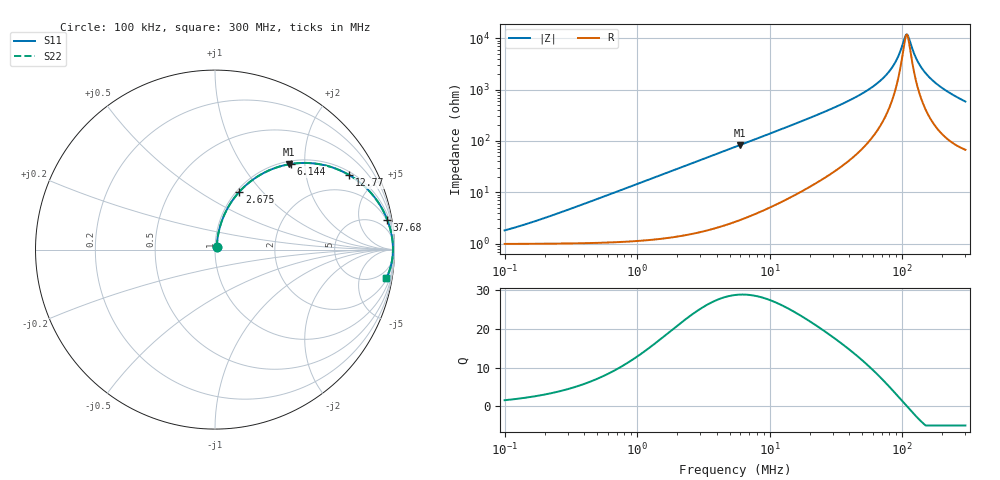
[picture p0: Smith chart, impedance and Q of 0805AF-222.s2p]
# MHz  S  MA  R  50
!Freq  MagS11  AngS11  MagS21  AngS21  MagS12  AngS12  MagS22  AngS22
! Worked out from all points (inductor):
!   801 points, 100 kHz to 300 MHz, reference 50 ohm
!   read as one part in series: L = 2.37 uH near 201.7 kHz
!   highest Q = 28.9 at 5.962 MHz (marker M1), where L = 2.21 uH
!   self-resonance near 107.9 MHz
!   S11 on the Smith chart (normalised r, x): 100 kHz: 1.02, +0.03; 2.675 MHz: 1.03, +0.76; 6.144 MHz: 1.06, +1.71; 12.77 MHz: 1.14, +3.52; 37.68 MHz: 2, +11; 300 MHz: 2, -12
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0.1  0.01791 56.1  0.9901 -0.9  0.9901 -0.9  0.01791 56.1
0.3829105  0.05666 76.6  0.9884 -3.2  0.9884 -3.2  0.05666 76.6
1.451587  0.2013 75.0  0.9677 -11.6  0.9677 -11.6  0.2013 75.0
2.674748  0.3487 67.2  0.9228 -20.4  0.9228 -20.4  0.3487 67.2
5.502866  0.5981 51.3  0.7809 -36.7  0.7809 -36.7  0.5981 51.3
5.96212  0.6275 49.2  0.7572 -38.8  0.7572 -38.8  0.6275 49.2
6.144056  0.6384 48.4  0.7479 -39.6  0.7479 -39.6  0.6384 48.4
8.724824  0.7568 38.8  0.6274 -49.1  0.6274 -49.1  0.7568 38.8
12.7677  0.8557 29.0  0.4854 -58.8  0.4854 -58.8  0.8557 29.0
20.86098  0.9328 18.6  0.3198 -68.7  0.3198 -68.7  0.9328 18.6
37.67659  0.9742 9.8  0.1711 -76.4  0.1711 -76.4  0.9742 9.8
59.14089  0.9868 5.1  0.08917 -79.0  0.08917 -79.0  0.9868 5.1
79.08254  0.9905 2.6  0.04531 -76.6  0.04531 -76.6  0.9905 2.6
90.08443  0.9913 1.5  0.02719 -70.6  0.02719 -70.6  0.9913 1.5
104.694  0.9916 0.3  0.009627 -29.5  0.009627 -29.5  0.9916 0.3
108.9752  0.9916 -0.0  0.008423 5.5  0.008423 5.5  0.9916 -0.0
112.3006  0.9916 -0.3  0.009799 30.5  0.009799 30.5  0.9916 -0.3
122.8982  0.9913 -1.0  0.01965 63.1  0.01965 63.1  0.9913 -1.0
130.5131  0.9909 -1.5  0.02761 70.1  0.02761 70.1  0.9909 -1.5
154.7495  0.9893 -2.9  0.05178 76.6  0.05178 76.6  0.9893 -2.9
204.8663  0.9837 -5.4  0.09553 77.4  0.09553 77.4  0.9837 -5.4
300  0.9673 -9.5  0.1657 73.9  0.1657 73.9  0.9673 -9.5
